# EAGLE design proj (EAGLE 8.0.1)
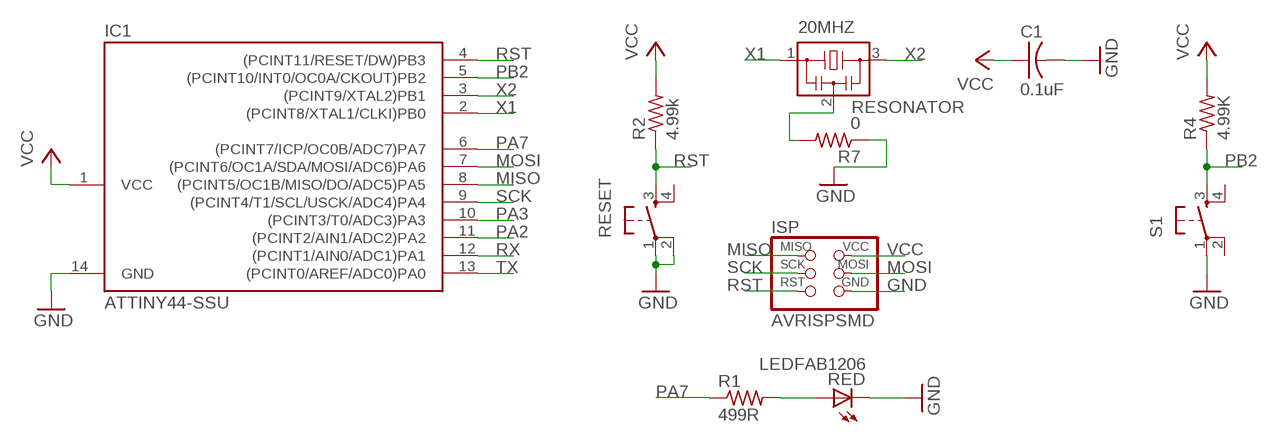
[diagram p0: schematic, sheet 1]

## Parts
20MHZ  RESONATOR  [EFOBM]
C1  0.1uF  CAP-US1206K  [C1206K]
IC1  ATTINY44-SSU  [SOIC14]
ISP  AVRISPSMD  [2X03SMD]
R1  499R  RES-US1206FAB  [R1206FAB]
R2  4.99k  RES-US1206FAB  [R1206FAB]
R4  4.99K  RES-US1206FAB  [R1206FAB]
R7  0  RES-US1206FAB  [R1206FAB]
RED  LEDFAB1206  [LED1206FAB]
RESET  6MM_SWITCH6MM_SWITCH  [6MM_SWITCH]
S1  6MM_SWITCH6MM_SWITCH  [6MM_SWITCH]

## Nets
GND: C1.2 IC1.14(GND) ISP.6(GND) R7.1 RED.2(C) RESET.1(P) RESET.2(P1) S1.1(P)
MISO: IC1.8((PCINT5/OC1B/MISO/DO/ADC5)PA5) ISP.1(MISO)
MOSI: IC1.7((PCINT6/OC1A/SDA/MOSI/ADC6)PA6) ISP.4(MOSI)
N$1: R1.2 RED.1(A)
N$2: 20MHZ.2 R7.2
PA2: IC1.11((PCINT2/AIN1/ADC2)PA2)
PA3: IC1.10((PCINT3/T0/ADC3)PA3)
PA7: IC1.6((PCINT7/ICP/OC0B/ADC7)PA7) R1.1
PB2: IC1.5((PCINT10/INT0/OC0A/CKOUT)PB2) R4.1 S1.3(S)
RST: IC1.4((PCINT11/RESET/DW)PB3) ISP.5(RST) R2.1 RESET.3(S)
RX: IC1.12((PCINT1/AIN0/ADC1)PA1)
SCK: IC1.9((PCINT4/T1/SCL/USCK/ADC4)PA4) ISP.3(SCK)
TX: IC1.13((PCINT0/AREF/ADC0)PA0)
VCC: C1.1 IC1.1(VCC) ISP.2(VCC) R2.2 R4.2
X1: 20MHZ.1 IC1.2((PCINT8/XTAL1/CLKI)PB0)
X2: 20MHZ.3 IC1.3((PCINT9/XTAL2)PB1)
Unconnected: RESET.4(S1) S1.2(P1) S1.4(S1)

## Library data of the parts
20MHZ = fab:RESONATOR
C1 = fab:CAP-US
IC1 = fab:ATTINY44
ISP = fab:AVRISP
R1 R2 R4 R7 = fab:RES-US: Resistor (US Symbol)
RED = fab:LED: LED
RESET S1 = fab:6MM_SWITCH: OMRON SWITCH

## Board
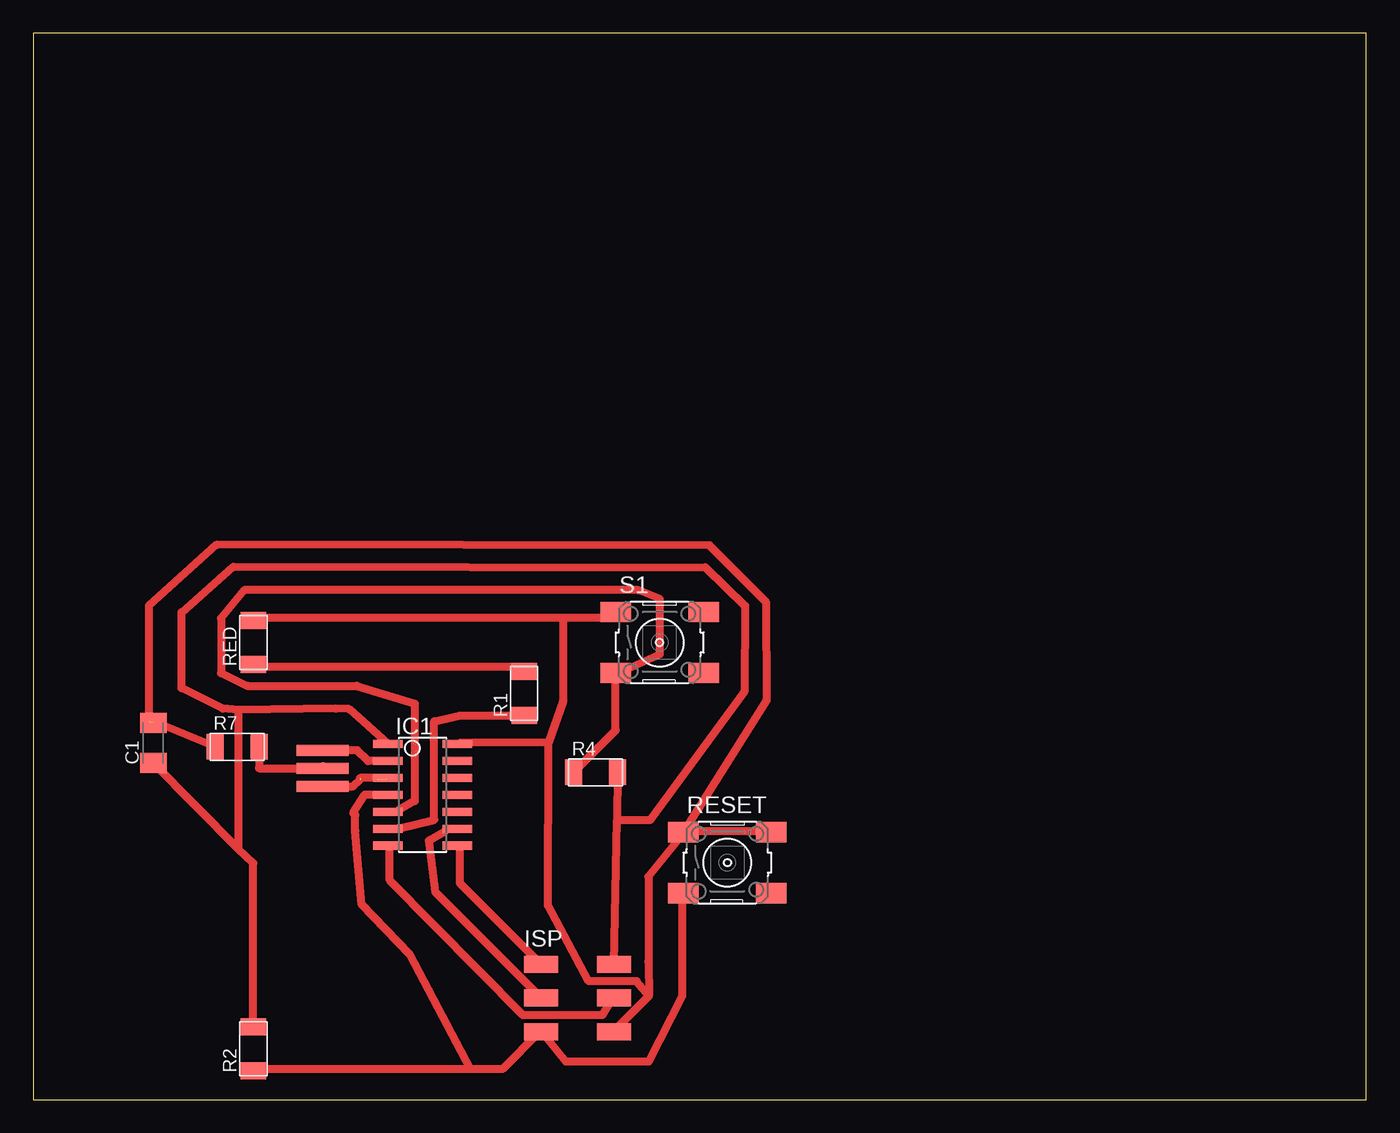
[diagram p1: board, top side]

Size 100 x 80 mm. Coordinates in mm from the lower left corner, seen from the top.
Outline: 0,0 100,0 100,80 0,80 0,0
Copper layers (1*16): Top 0.035mm / dielectric 1.5mm / Bottom 0.035mm
Design rules "default": minimum track width 10mil, minimum drill 24mil, track to track 8mil, track to pad 8mil, pad to pad 8mil, via to via 8mil, smd to smd 8mil, copper to edge 40mil, drill to drill 8mil, minimum pad ring 10mil, minimum via ring 8mil, stop-mask expansion 4mil, vias tented up to drill 0mil, thermal gap 10mil

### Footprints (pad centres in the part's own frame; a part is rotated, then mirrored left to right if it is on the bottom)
EFOBM = smd 0.8 x 3.9: 1 -1.35,0; 2 0,0; 3 1.35,0
C1206K = smd 1.5 x 2: 1 -1.5,0; 2 1.5,0
SOIC14 = smd 0.61 x 2.21: 1 -3.81,-2.603; 2 -2.54,-2.603; 3 -1.27,-2.603; 4 0,-2.603; 5 1.27,-2.603; 6 2.54,-2.603; 7 3.81,-2.603; 8 3.81,2.603; 9 2.54,2.603; 10 1.27,2.603; 11 0,2.603; 12 -1.27,2.603; 13 -2.54,2.603; 14 -3.81,2.603
2X03SMD = smd 2.54 x 1.27: 1 -2.54,2.54; 2 2.92,2.54; 3 -2.54,0; 4 2.92,0; 5 -2.54,-2.54; 6 2.92,-2.54
R1206FAB = smd 1.27 x 1.905: 1 -1.651,0; 2 1.651,0
LED1206FAB = smd 1.27 x 1.905: 1 -1.651,0; 2 1.651,0
6MM_SWITCH = smd 2.286 x 1.524: 1 -3.302,2.286; 2 3.302,2.286; 3 -3.302,-2.286; 4 3.302,-2.286

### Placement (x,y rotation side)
20MHZ  21.71,24.85 270 top
C1  9.01,26.74 90 top
IC1  29.21,22.86 270 top
ISP  40.64,7.62 0 top
R1  36.83,30.48 90 top
R2  16.51,3.81 90 top
R4  42.18,24.55 0 top
R7  15.29,26.47 0 top
RED  16.51,34.29 90 top
RESET  52.07,17.78 0 top
S1  46.99,34.29 0 top

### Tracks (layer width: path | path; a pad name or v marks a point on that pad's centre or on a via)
GND  (1 unrouted)
  Top 0.254: 43.2,36.12 43.66,36.58 S1.1 | 16.69,36.12 RED.2 | 32,26.75 IC1.14 | 48.92,20.12 RESET.1 48.69,19.89 | 55.32,20.12 RESET.2 | 43.66,5.26 ISP.6
  Top 0.61: 43.2,36.12 39.73,36.12 | 39.73,36.12 16.69,36.12 | 38.66,26.8 32,26.75 | 38.66,26.8 39.73,29.87 39.73,36.12 | 55.32,20.12 48.92,20.12 | 46.18,7.77 46.14,10.34 46.14,16.74 48.69,19.89 | 46.18,7.77 43.66,5.26 | 8.67,28.32 8.67,37.03 13.77,41.63 50.74,41.58 54.99,37.28 55.04,30.02 RESET.1 | 38.66,26.8 38.6,14.55 41.67,8.89 45.26,8.89 46.18,7.77 | R7.1 9.09,28.32 C1.2
MISO
  Top 0.254: 32,18.97 IC1.8 | 37.95,10.29 ISP.1
  Top 0.61: 32,18.97 32,16.23 37.95,10.29
MOSI
  Top 0.254: 26.75,18.97 IC1.7 | 43.43,7.54 ISP.4
  Top 0.61: 26.75,18.97 26.75,16.46 36.73,6.33 42.67,6.33 43.43,7.54
N$1
  Top 0.254: 36.58,32.46 36.8,32.23 R1.2 | 16.69,32.46 RED.1
  Top 0.61: 36.58,32.46 16.69,32.46
N$2
  Top 0.61: 21.71,25.02 20MHZ.2 16.94,24.85 R7.2
PA7
  Top 0.254: 27.43,20.34 26.75,20.34 IC1.6 | 36.8,28.8 R1.1
  Top 0.61: 36.8,28.8 32,28.8 30.07,28.38 30.07,20.99 27.43,20.34
PB2
  Top 0.254: 40.7,24.57 R4.1 | 27.43,21.72 26.75,21.72 IC1.5 | S1.3 43.89,32
  Top 0.61: 40.65,24.57 40.7,24.57 | 27.43,21.72 28.62,22.4 28.62,29.7 24.27,31.05 16.05,31.05 14.09,32 14.09,36.13 15.83,38.22 45.38,38.22 47.01,37.54 47.01,33.43 43.89,32 | R4.1 43.69,27.71 S1.3
RST
  Top 0.254: 16.69,2.29 R2.1 | 37.95,5.03 ISP.5 38.18,5.03 | 48.69,15.32 RESET.3
  Top 0.61: 32.82,2.29 35.2,2.29 37.95,5.03 | 32.82,2.29 16.69,2.29 | 32.82,2.29 28.27,10.86 24.65,14.63 24.15,20.17 24.15,21.35 24,21.5 24.86,22.86 IC1.4 | 48.69,15.32 48.69,7.77 46.18,2.87 39.94,2.87 38.18,5.03
SCK
  Top 0.254: 30.86,20.12 31.77,20.12 IC1.9
  Top 0.61: 30.86,20.12 29.68,19.43 30.18,15.54 ISP.3
VCC
  Top 0.254: 43.86,24.5 R4.2 | 43.43,10.29 ISP.2 | 16.69,5.49 R2.2 | 26.52,26.52 IC1.1
  Top 0.61: 43.8,20.97 46.32,21 53.36,30.58 53.41,37.03 50.41,39.93 15,39.98 11.13,36.55 11.13,30.88 14.22,29.34 15.35,29.24 | 15.35,29.24 22.68,29.34 23.69,29.29 IC1.1 | R2.2 16.51,17.74 15.38,18.82 | 15.38,18.82 C1.1 | 15.35,29.24 15.38,18.82 | R4.2 43.8,20.97 | ISP.2 43.8,20.97
X1
  Top 0.254: 25.83,25.38 26.52,25.38 IC1.2
  Top 0.61: 20MHZ.1 24.3,26.2 25.1,25.4 IC1.2
X2  (3 unrouted)
  Top 0.254: 26.52,24 IC1.3
  Top 0.61: 20MHZ.3 24,23.5 24.5,24 | IC1.3 24.5,24.13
